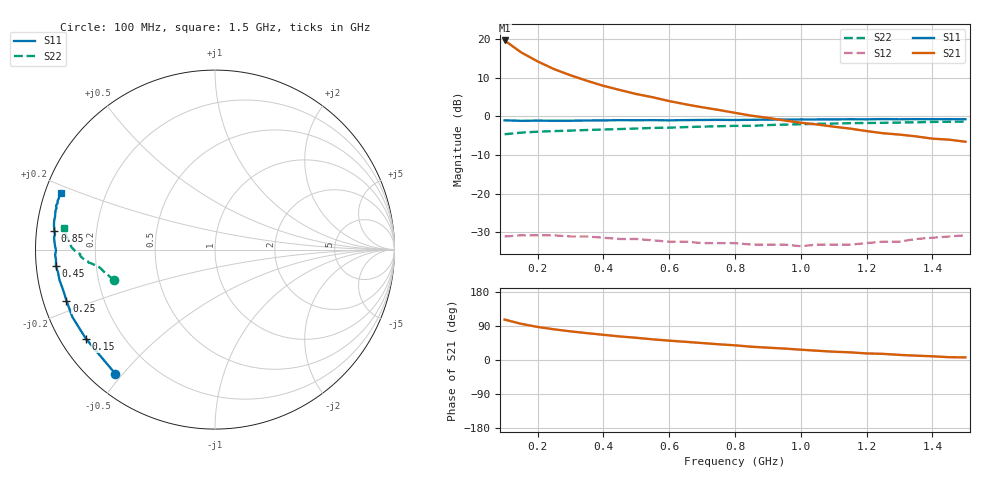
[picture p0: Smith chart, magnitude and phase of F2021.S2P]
!  POLYFET RF DEVICES
!  F2021
!  S PARAMETERS
!  VDS=28V, IDQ=600mA
!Date: 10/21/91
# MHZ S MA R 50
!FREQ-MHZ MAG[S11] ANG[S11] MAG[S21] ANG[S21] MAG[S12] ANG[S12] MAG[S22] ANG[S22]
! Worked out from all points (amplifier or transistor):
!   29 points, 100 MHz to 1.5 GHz, reference 50 ohm
!   highest |S21| = 19.6 dB at 100 MHz (marker M1)
!   |S21| within 3 dB of that: start of sweep to 148.9 MHz
!   unconditionally stable (mu >= 1): 599.6 MHz to end of sweep
!   at 300 MHz: K = 0.44, MSG = 20.8 dB, |S12| = -31.1 dB
!   at 800 MHz: K = 1.28, MAG = 13.7 dB, |S12| = -32.8 dB
!   at 1.5 GHz: K = 1.46, MAG = 8.1 dB, |S12| = -30.8 dB
!   S11 on the Smith chart (normalised r, x): 100 MHz: 0.07, -0.48; 150 MHz: 0.07, -0.31; 250 MHz: 0.07, -0.17; 450 MHz: 0.06, -0.05; 850 MHz: 0.05, +0.06; 1.5 GHz: 0.05, +0.18
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100  0.887 -128.8  9.538 106.7  0.028 22.4  0.586 -162.9
150  0.874 -145.3  6.701 95.5  0.029 14.0  0.615 -166.9
200  0.879 -154.7  5.123 87.2  0.029 8.6  0.632 -168.9
250  0.875 -161.1  4.07 81.0  0.029 5.7  0.644 -170.5
300  0.876 -165.6  3.388 75.6  0.028 4.1  0.653 -171.4
350  0.883 -168.9  2.876 70.9  0.028 2.4  0.665 -172.1
400  0.884 -171.9  2.474 66.5  0.027 1.7  0.674 -172.6
450  0.891 -174.1  2.187 62.1  0.026 1.2  0.684 -173.2
500  0.888 -176.1  1.938 58.6  0.026 1.4  0.695 -173.7
550  0.891 -178.2  1.761 54.5  0.025 1.5  0.707 -174.1
600  0.886 -179.8  1.572 51.0  0.024 3.0  0.713 -174.8
700  0.896 177.1  1.308 44.8  0.023 5.9  0.735 -176.0
800  0.895 174.6  1.108 38.7  0.023 8.6  0.752 -177.4
850  0.901 173.3  1.018 35.0  0.022 11.1  0.752 -178.1
950  0.909 170.8  0.883 30.2  0.022 16.5  0.781 -179.5
1000  0.91 169.7  0.826 27.2  0.021 18.4  0.789 179.8
1050  0.91 168.3  0.783 24.4  0.022 20.2  0.8 179.1
1150  0.915 166.2  0.693 20.2  0.022 27.6  0.815 177.3
1200  0.913 165.3  0.644 17.3  0.023 30.6  0.819 176.5
1300  0.914 163.6  0.58 13.5  0.024 35.6  0.83 174.8
1350  0.918 162.7  0.55 11.5  0.026 37.9  0.836 174.2
1500  0.915 160.0  0.469 6.9  0.029 41.3  0.852 171.8
